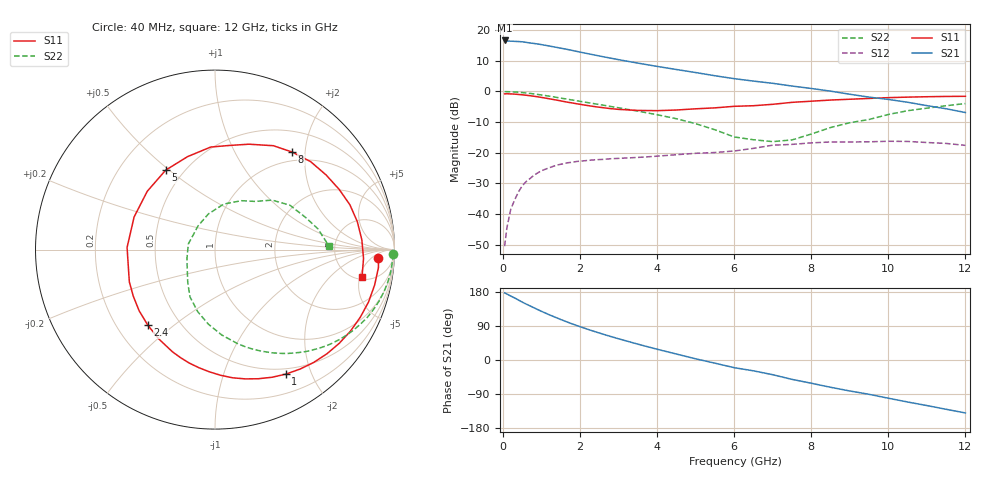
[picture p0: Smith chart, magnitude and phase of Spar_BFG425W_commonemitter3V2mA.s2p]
! Filename: 32bfg425.001
! BFG425W Field C1
! V1=8.039E-001V,V2=3.000E+000V, I1=2.337E-005A, I2=2.000E-003A
# GHz  S  MA  R 50
!  S11  S21  S12  S22
!Freq(GHz)  Mag  Ang  Mag  Ang  Mag  Ang  Mag  Ang
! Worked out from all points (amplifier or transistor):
!   44 points, 40 MHz to 12 GHz, reference 50 ohm
!   highest |S21| = 16.6 dB at 40 MHz (marker M1)
!   |S21| within 3 dB of that: start of sweep to 1.698 GHz
!   unconditionally stable (mu >= 1): 3.099 GHz to end of sweep
!   at 700 MHz: K = 0.18, MSG = 22.1 dB, |S12| = -28.4 dB
!   at 2.4 GHz: K = 0.72, MSG = 17.0 dB, |S12| = -22.3 dB
!   at 12 GHz: K = 1.79, MAG = 0.2 dB, |S12| = -17.6 dB
!   S11 on the Smith chart (normalised r, x): 40 MHz: 16, -9; 1 GHz: 0.43, -1.64; 2.4 GHz: 0.33, -0.41; 5 GHz: 0.40, +0.49; 8 GHz: 0.84, +1.75; 12 GHz: 5.48, -5.44
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0.04  0.912 -3.0  6.781 177.1  0.003 68.8  0.992 -1.4
0.1  0.916 -6.3  6.638 174.2  0.006 84.5  0.991 -3.6
0.2  0.911 -12.5  6.604 168.7  0.012 80.6  0.987 -7.1
0.5  0.881 -31.0  6.441 152.7  0.029 69.2  0.958 -17.5
0.8  0.835 -48.9  6.054 137.8  0.043 58.1  0.911 -27.0
1  0.798 -60.4  5.799 128.3  0.051 51.4  0.875 -33.0
1.2  0.759 -71.4  5.502 119.4  0.057 45.3  0.837 -38.5
1.5  0.701 -87.4  5.074 106.8  0.065 37.1  0.779 -45.9
1.8  0.648 -102.9  4.655 95.1  0.07 30.2  0.724 -52.7
2.2  0.588 -122.2  4.131 81.0  0.075 22.7  0.657 -61.1
2.4  0.563 -131.8  3.899 74.3  0.077 19.6  0.626 -64.9
3  0.51 -159.4  3.296 55.9  0.081 12.1  0.541 -76.2
3.5  0.49 178.6  2.896 41.8  0.084 7.5  0.477 -85.5
4  0.486 158.0  2.559 28.3  0.088 3.4  0.417 -95.1
4.5  0.498 139.3  2.278 15.7  0.093 -0.3  0.359 -105.5
5  0.521 121.8  2.032 3.1  0.098 -5.6  0.298 -117.9
6  0.572 92.4  1.615 -20.3  0.107 -15.7  0.181 -149.0
6.5  0.585 82.5  1.475 -28.6  0.118 -13.6  0.163 -163.2
8  0.693 51.7  1.118 -61.3  0.145 -37.7  0.202 100.6
8.5  0.724 42.6  1.011 -72.0  0.15 -46.8  0.258 79.1
10.5  0.808 11.1  0.666 -110.8  0.153 -81.6  0.485 30.7
12  0.833 -10.5  0.453 -139.7  0.132 -113.1  0.635 1.8
